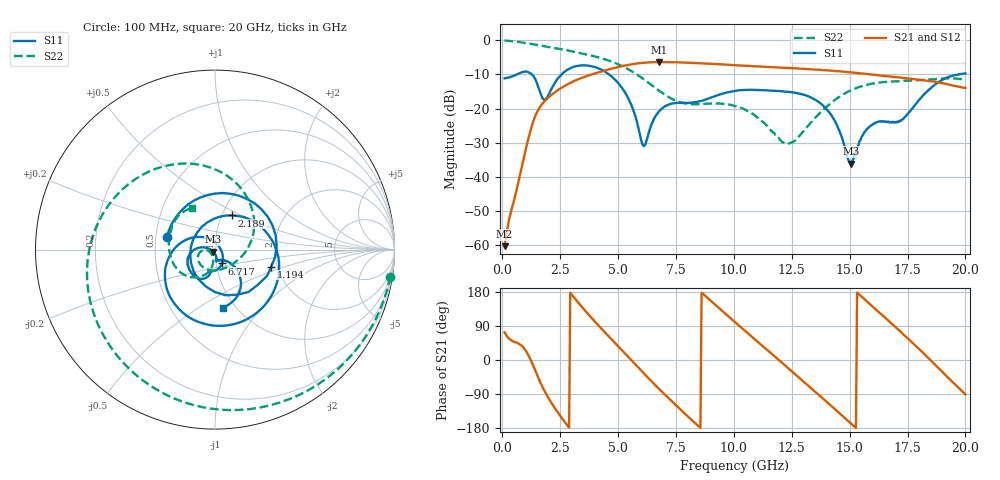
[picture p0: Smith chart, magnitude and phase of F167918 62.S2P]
!  2-Port S-parameters saved by WinCal
! VAR MeasName=S-Parameters (CALIBRATED_DATA) read from VNA (N5242A)
! VAR MeasDate=2016-11-22 10:27:54
! VAR NAME=F167918 62
! VAR FILENAME=F167918 62.S2P
! VAR DATE=2016-11-22 10:27:54
! VAR PHYS_PORTS=1,2
# Hz S DB R 50
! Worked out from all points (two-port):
!   401 points, 100 MHz to 20 GHz, reference 50 ohm
!   highest |S21| = -6.40 dB at 6.766 GHz (marker M1); lowest = -60.2 dB at 100 MHz (marker M2)
!   |S21| within 3 dB of the highest: 4.156 GHz to 14.99 GHz (10.83 GHz wide, 113 % of centre)
!   lowest |S11| = -36.1 dB at 15.07 GHz (marker M3), VSWR 1.03, Z = 49 - j1.21 ohm
!   |S11| at or under -10 dB: start of sweep to 633.9 MHz; 1.272 GHz to 2.567 GHz (1.295 GHz wide, 67.5 % of centre); 4.606 GHz to 19.73 GHz (15.12 GHz wide, 124 % of centre)
!   |S22| runs from -30.3 to -0.1 dB; largest |S21 - S12| = 0.0048
!   S11 on the Smith chart (normalised r, x): 100 MHz: 0.57, +0.09; 1.194 GHz: 1.86, -0.39; 2.189 GHz: 1.12, +0.44; 6.717 GHz: 1.07, -0.17; 20 GHz: 0.88, -0.63
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1e8  -11.16 165.3  -60.22 72.7  -61.13 77.9  -0.10 -8.8
6.97e8  -9.82 74.5  -41.51 43.8  -41.56 43.7  -0.53 -56.2
1.1945e9  -9.69 -16.7  -27.06 4.4  -27.10 4.7  -1.05 -91.2
1.692e9  -16.32 -151.1  -18.94 -65.6  -18.93 -65.4  -1.65 -121.4
2.1895e9  -13.45 63.5  -15.64 -119.6  -15.64 -119.4  -2.23 -147.5
2.7865e9  -8.75 -11.9  -13.01 -170.7  -13.00 -170.4  -2.96 -175.5
3.43325e9  -7.38 -69.2  -11.02 140.3  -10.98 140.6  -3.86 156.8
4.32875e9  -8.79 -133.5  -9.06 79.7  -8.99 79.5  -5.39 119.2
5.075e9  -13.12 177.1  -7.74 31.4  -7.73 31.1  -7.26 85.8
6.11975e9  -30.97 31.6  -6.61 -35.6  -6.62 -35.8  -11.49 35.0
6.71675e9  -21.26 -63.2  -6.41 -73.1  -6.41 -73.0  -14.52 5.1
6.7665e9  -20.87 -66.4  -6.40 -76.0  -6.42 -76.1  -14.77 2.4
8.40825e9  -18.06 -102.0  -6.72 -171.0  -6.70 -171.0  -18.72 -80.7
1.005e10  -14.81 -116.0  -7.30 99.8  -7.29 99.8  -19.25 -149.4
1.228875e10  -15.11 -147.7  -8.11 -18.3  -8.09 -18.5  -30.29 -144.6
1.338325e10  -16.98 -170.2  -8.53 -76.8  -8.51 -76.8  -23.69 -98.9
1.427875e10  -22.66 169.7  -8.95 -125.1  -8.97 -125.2  -17.97 -105.9
1.507475e10  -36.07 -128.0  -9.43 -168.3  -9.44 -168.5  -14.66 -123.1
1.577125e10  -25.90 -80.3  -9.92 153.3  -9.93 153.5  -13.06 -141.7
1.67165e10  -24.04 -79.4  -10.58 101.7  -10.63 101.9  -12.18 -164.7
1.83085e10  -15.27 -43.3  -11.86 10.8  -11.77 11.0  -11.54 162.7
2e10  -9.72 -82.4  -13.94 -90.8  -13.82 -90.8  -11.62 118.6
